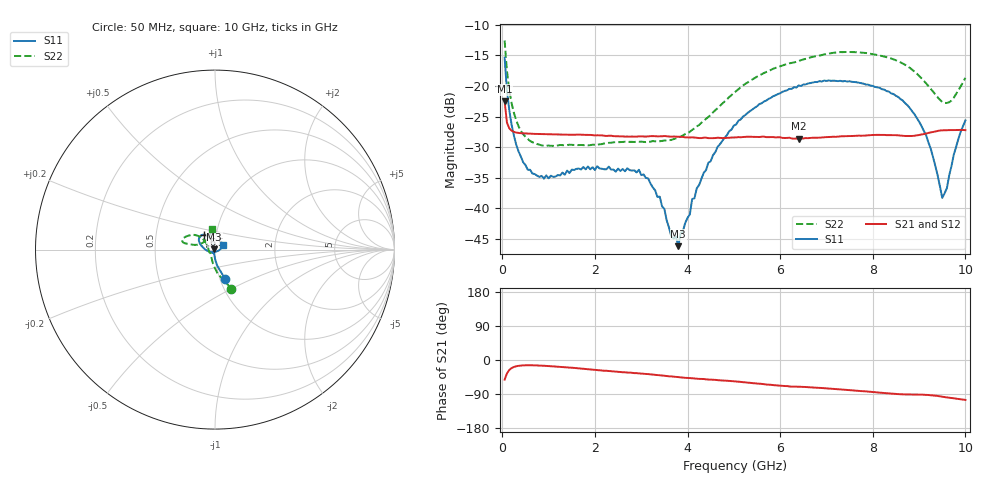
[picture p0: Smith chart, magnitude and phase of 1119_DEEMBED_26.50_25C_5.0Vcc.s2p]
!Hittite Microwave Corp.
!Digital Attenuator/PhaseShifter Rev 1.4.0
!Filename: C:\DATA\DATA\1119_DEEMBED_26.50_25C_5.0Vcc.s2p
!VNA ID: Agilent Technologies,N5224A,MY51441122,A.10.45.03
!Device type:
!2 Port Calibration.
!Temp(C): 25
!Lot Number:
!Serial Number:
!Operator:
!Misc:
!Attenuator:  26.500
# GHZ S DB R 50.0
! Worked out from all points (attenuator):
!   200 points, 50 MHz to 10 GHz, reference 50 ohm
!   highest |S21| = -22.50 dB at 50 MHz (marker M1); lowest = -28.6 dB at 6.4 GHz (marker M2)
!   lowest |S11| = -46.2 dB at 3.8 GHz (marker M3), VSWR 1.01, Z = 49.5 + j0.107 ohm
!   |S11| at or under -10 dB: start of sweep to end of sweep
!   |S22| runs from -29.8 to -12.6 dB; largest |S21 - S12| = 0.00012
!   S11 on the Smith chart (normalised r, x): 50 MHz: 1.06, -0.35; 6.5 GHz: 0.87, +0.15; 10 GHz: 1.10, +0.05
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0.05  -15.37 -71.2  -22.50 -51.8  -22.51 -51.8  -12.56 -67.3
0.1  -20.70 -81.7  -25.96 -35.5  -25.97 -35.5  -17.51 -83.9
0.2  -26.29 -90.4  -27.31 -21.4  -27.31 -21.3  -22.79 -100.5
0.55  -33.69 -104.8  -27.79 -13.8  -27.79 -13.8  -28.66 -126.3
0.9  -35.15 -112.0  -27.87 -15.2  -27.87 -15.3  -29.77 -135.7
1.75  -33.25 -121.4  -27.98 -23.2  -27.98 -23.3  -29.67 -140.7
2.95  -33.69 -113.8  -28.23 -35.1  -28.24 -35.2  -29.12 -159.9
3.4  -38.09 -126.4  -28.22 -40.2  -28.23 -40.2  -29.03 -173.5
3.65  -44.56 -150.1  -28.29 -43.3  -28.30 -43.3  -28.81 177.4
3.8  -46.18 167.3  -28.30 -45.3  -28.30 -45.4  -28.45 170.6
4.1  -38.47 113.5  -28.39 -48.3  -28.40 -48.4  -27.18 158.3
4.45  -32.53 100.0  -28.53 -51.6  -28.55 -51.8  -25.05 146.4
5.05  -26.29 105.7  -28.40 -56.6  -28.41 -56.7  -20.83 138.8
6.4  -19.91 124.3  -28.62 -70.6  -28.63 -70.6  -15.93 149.9
6.5  -19.76 126.0  -28.58 -70.9  -28.58 -70.9  -15.67 151.5
6.7  -19.45 129.7  -28.46 -72.5  -28.48 -72.5  -15.24 153.9
8.35  -20.93 158.6  -28.03 -88.1  -28.03 -88.1  -15.40 168.1
8.75  -23.15 169.1  -28.17 -90.9  -28.17 -91.0  -16.78 168.1
9.15  -28.01 -166.8  -27.77 -91.9  -27.79 -91.9  -19.55 165.4
9.5  -38.29 -92.1  -27.25 -96.9  -27.27 -96.9  -22.61 144.0
9.7  -33.08 -12.0  -27.21 -100.3  -27.22 -100.3  -22.39 119.9
10  -25.63 26.9  -27.22 -105.4  -27.24 -105.3  -18.67 98.5
